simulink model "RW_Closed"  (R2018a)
settings: Solver=ode8  StartTime=0.0  StopTime=1000  FixedStep=Ts  MaxStep=0.5  RelTol=1e-3  EnableMultiTasking=on
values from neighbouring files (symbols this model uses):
  d2r = pi/180    (= 0.0174532925199)    [run.m]    (also in runf.m; orbitic.m; Quan.m)
  ini = [wb0; atto; Hco]    [run.m]
  Kq1 = I22*ww^2 - 3*wo2*(I11-I33)    [run.m]
  Kq2 = 2*I22*zet*ww    [run.m]
  Kqi = 0.0005    [run.m]
  Kr1 = (0.1*I11*I33*zet^2/Hy0) - sqrt( ((0.01^zet^4*I11^2*I33^2)/Hy0^2)+(4*I11*I33*zet^2) )    [run.m]
  Kr2 = 0.05*Kr1    [run.m]
  Kr3 = 0.04*zet*(Kr2-Hy0) * sqrt(abs(Hy0/(I11*I33)))    [run.m]
  nt = 7    [run.m]    (also in runf.m)
  r2d = 180/pi    (= 57.2957795131)    [pl.m]    (also in run.m; plf.m; runf.m; pl2.m)
  Ts = 0.001    [run.m]    (also in runf.m = 0.0005)
undefined symbols (not defined in the file or in its folder): DiscIntNeverNeededParam, NonLin_Vehi_Dynamics, RW_Steering
libraries: simulink x3

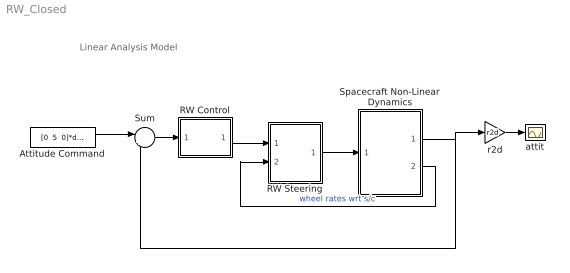
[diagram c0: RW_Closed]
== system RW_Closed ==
  note: Linear Analysis Model
  Attitude Command : Constant  Value="[0  5  0]*d2r"
  RW Control : Subsystem
  RW Steering : Subsystem
  Spacecraft Non-Linear Dynamics : Subsystem
  Sum : Sum  Inputs=|+-
  attit : Scope
  r2d : Gain  Gain=r2d
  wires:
  Spacecraft Non-Linear Dynamics/2(wr) -> RW Steering/2(wr(1))  "wheel rates wrt s/c"
  Spacecraft Non-Linear Dynamics/1(att-lv) -> r2d/1, Sum/2
  RW Steering/1(Twi) -> Spacecraft Non-Linear Dynamics/1(Twi)
  RW Control/1(Tc) -> RW Steering/1(Trwc)
  Sum/1 -> RW Control/1(atti)
  Attitude Command/1 -> Sum/1
  r2d/1 -> attit/1

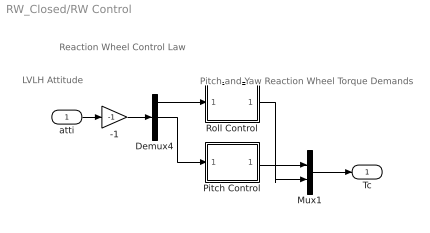
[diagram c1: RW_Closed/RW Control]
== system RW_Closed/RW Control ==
  note: Reaction Wheel Control Law
  note: LVLH Attitude
  note: Pitch and Yaw Reaction Wheel Torque Demands
  atti : Inport
  -1 : Gain  Gain=-1
  Demux4 : Demux  Outputs=3
  Mux1 : Mux  Inputs=2
  Pitch Control : Subsystem
  Roll Control : Subsystem
  Tc : Outport
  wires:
  Mux1/1 -> Tc/1
  Roll Control/1(Tcz) -> Mux1/2
  -1/1 -> Demux4/1
  atti/1 -> -1/1
  Demux4/2 -> Pitch Control/1(the)
  Pitch Control/1(Tcy) -> Mux1/1
  Demux4/1 -> Roll Control/1(phi)

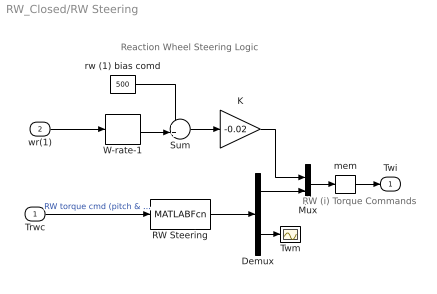
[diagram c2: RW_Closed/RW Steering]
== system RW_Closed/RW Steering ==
  note: Reaction Wheel Steering Logic
  note: RW (i) Torque Commands
  Trwc : Inport
  wr(1) : Inport  Port=2
  Demux : Demux  Outputs=[2, 1]
  K : Gain  Gain=-0.02
  Mux : Mux  Inputs=[1,2]
  RW Steering : MATLABFcn  MATLABFcn=RW_Steering( u(1:2) )  OutputDimensions=3
  Sum : Sum  Inputs=++|
  Twm : Scope
  W-rate-1 : Selector  InputPortWidth=3  IndexOptions=Index vector (dialog)  Indices=[1]  OutputSizes=1
  mem : Memory
  rw (1) bias comd : Constant  Value=500
  Twi : Outport
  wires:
  mem/1 -> Twi/1
  K/1 -> Mux/1
  W-rate-1/1 -> Sum/2
  rw (1) bias comd/1 -> Sum/1
  Sum/1 -> K/1
  wr(1)/1 -> W-rate-1/1
  Mux/1 -> mem/1
  Trwc/1 -> RW Steering/1  "RW torque cmd (pitch & yaw)"
  RW Steering/1 -> Demux/1
  Demux/1 -> Mux/2
  Demux/2 -> Twm/1

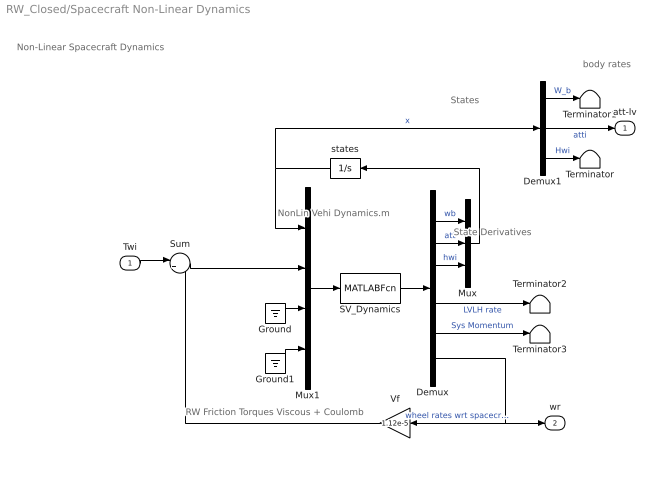
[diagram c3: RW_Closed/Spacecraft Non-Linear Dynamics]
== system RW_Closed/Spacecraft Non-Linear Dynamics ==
  note: NonLin Vehi Dynamics.m
  note: Non-Linear Spacecraft Dynamics
  note: RW Friction Torques Viscous + Coulomb
  note: States
  note: body rates
  note: State Derivatives
  Twi : Inport
  Demux : Demux  Outputs="[3,3,3,  3,3,3]"
  Demux1 : Demux  Outputs=[3,3,3]
  Ground : Ground
  Ground1 : Ground
  Mux : Mux  Inputs=[3,3,3]
  Mux1 : Mux  Inputs=[9,3, nt, 3]
  SV_Dynamics : MATLABFcn  MATLABFcn=NonLin_Vehi_Dynamics( u(1:9), u(10:12), u(13:12+nt), u(13+nt:15+nt) )  OutputDimensions=9+9
  Sum : Sum  Inputs=|+-
  Terminator{,1..3} (4 alike) : Terminator
  Vf : Gain  Gain=1.12e-5
  states : Integrator  InitialCondition=ini
  att-lv : Outport
  wr : Outport  Port=2
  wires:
  Ground1/1 -> Mux1/4
  Demux/5 -> Terminator3/1  "Sys Momentum"
  Demux/4 -> Terminator2/1  "LVLH rate"
  Demux1/1 -> Terminator1/1  "W_b"
  Demux1/3 -> Terminator/1  "Hwi"
  Mux/1 -> states/1
  Demux/3 -> Mux/3  "hwi"
  Demux/2 -> Mux/2  "att"
  Demux/1 -> Mux/1  "wb"
  Ground/1 -> Mux1/3
  Sum/1 -> Mux1/2
  Twi/1 -> Sum/1
  Vf/1 -> Sum/2
  states/1 -> Mux1/1, Demux1/1  "x"
  SV_Dynamics/1 -> Demux/1
  Mux1/1 -> SV_Dynamics/1
  Demux1/2 -> att-lv/1  "atti"
  Demux/6 -> Vf/1, wr/1  "wheel rates wrt spacecrft"

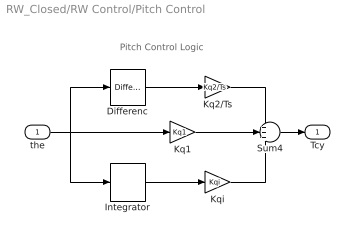
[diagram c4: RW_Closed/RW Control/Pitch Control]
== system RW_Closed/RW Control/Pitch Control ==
  note: Pitch Control Logic
  the : Inport
  Differenc : simulink/Discrete/Difference  ICPrevInput=0.0  InputProcessing=Inherited  OutMin=[]  OutMax=[]  OutDataType=sfix(16)  OutScaling=2^-10  DoSatur=off
  Integrator : DiscreteIntegrator  SampleTime=Ts  ICPrevOutput=DiscIntNeverNeededParam  ICPrevScaledInput=DiscIntNeverNeededParam
  Kq1 : Gain  Gain=Kq1
  Kq2/Ts : Gain  Gain=Kq2/Ts
  Kqi : Gain  Gain=Kqi
  Sum4 : Sum  Inputs=+++
  Tcy : Outport
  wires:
  Differenc/1 -> Kq2/Ts/1
  Integrator/1 -> Kqi/1
  Kqi/1 -> Sum4/3
  the/1 -> Differenc/1, Integrator/1, Kq1/1
  Kq2/Ts/1 -> Sum4/1
  Sum4/1 -> Tcy/1
  Kq1/1 -> Sum4/2

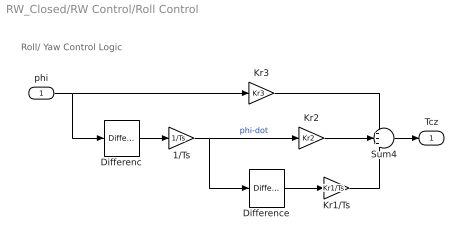
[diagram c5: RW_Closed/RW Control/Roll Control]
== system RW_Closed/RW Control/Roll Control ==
  note: Roll/ Yaw Control Logic
  phi : Inport
  1/Ts : Gain  Gain=1/Ts
  Differenc : simulink/Discrete/Difference  ICPrevInput=0.0  InputProcessing=Inherited  OutMin=[]  OutMax=[]  OutDataType=sfix(16)  OutScaling=2^-10  DoSatur=off
  Difference : simulink/Discrete/Difference  ICPrevInput=0.0  InputProcessing=Inherited  OutMin=[]  OutMax=[]  OutDataType=sfix(16)  OutScaling=2^-10  DoSatur=off
  Kr1/Ts : Gain  Gain=Kr1/Ts
  Kr2 : Gain  Gain=Kr2
  Kr3 : Gain  Gain=Kr3
  Sum4 : Sum  Inputs=+++
  Tcz : Outport
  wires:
  1/Ts/1 -> Difference/1, Kr2/1  "phi-dot"
  Differenc/1 -> 1/Ts/1
  Difference/1 -> Kr1/Ts/1
  Sum4/1 -> Tcz/1
  phi/1 -> Differenc/1, Kr3/1
  Kr1/Ts/1 -> Sum4/3
  Kr2/1 -> Sum4/2
  Kr3/1 -> Sum4/1
